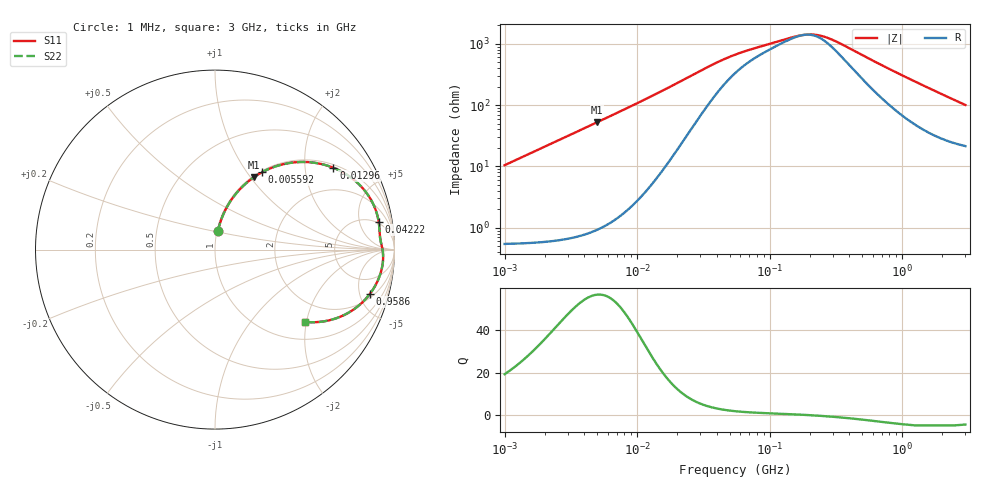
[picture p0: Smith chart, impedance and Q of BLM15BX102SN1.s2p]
! BLM15BX102SN1
# Hz S RI R 50
!Freq.(Hz) S11(Real) S11(Imag) S21(Real) S21(Imag) S12(Real) S12(Imag) S22(Real) S22(Imag)
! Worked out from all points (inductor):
!   401 points, 1 MHz to 3 GHz, reference 50 ohm
!   read as one part in series: L = 1.66 uH near 1.041 MHz
!   highest Q = 56.7 at 4.959 MHz (marker M1), where L = 1.67 uH
!   self-resonance near 183.5 MHz
!   S11 on the Smith chart (normalised r, x): 1 MHz: 1.01, +0.21; 5.592 MHz: 1.02, +1.18; 12.96 MHz: 1.10, +2.82; 42.22 MHz: 5, +10; 958.6 MHz: 2.45, -6.22; 3 GHz: 1.43, -1.96
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1000000  0.016 0.1021  0.984 -0.1021  0.984 -0.1021  0.016 0.1021
2182827  0.0545 0.2143  0.9455 -0.2143  0.9455 -0.2143  0.0545 0.2143
3823119  0.1428 0.3407  0.8572 -0.3407  0.8572 -0.3407  0.1428 0.3407
4959344  0.2175 0.4038  0.7825 -0.4038  0.7825 -0.4038  0.2175 0.4038
5592179  0.2608 0.4303  0.7392 -0.4303  0.7392 -0.4303  0.2608 0.4303
8686058  0.4616 0.4876  0.5384 -0.4876  0.5384 -0.4876  0.4616 0.4876
1.29622e7  0.6599 0.4558  0.3401 -0.4558  0.3401 -0.4558  0.6599 0.4558
1.461624e7  0.7121 0.431  0.2879 -0.431  0.2879 -0.431  0.7121 0.431
1.858443e7  0.7981 0.3678  0.2019 -0.3678  0.2019 -0.3678  0.7981 0.3678
2.362996e7  0.8571 0.2972  0.1429 -0.2972  0.1429 -0.2972  0.8571 0.2972
4.22235e7  0.9121 0.1534  0.0879 -0.1534  0.0879 -0.1534  0.9121 0.1534
5.477226e7  0.9164 0.1114  0.0836 -0.1114  0.0836 -0.1114  0.9164 0.1114
1.460522e8  0.9293 0.0199  0.0707 -0.0199  0.0707 -0.0199  0.9293 0.0199
2.094008e8  0.9351 -0.0125  0.0649 0.0125  0.0649 0.0125  0.9351 -0.0125
2.457655e8  0.9365 -0.0288  0.0635 0.0288  0.0635 0.0288  0.9365 -0.0288
3.002264e8  0.9366 -0.0513  0.0634 0.0513  0.0634 0.0513  0.9366 -0.0513
5.154121e8  0.924 -0.1266  0.076 0.1266  0.076 0.1266  0.924 -0.1266
8.005644e8  0.8889 -0.2079  0.1111 0.2079  0.1111 0.2079  0.8889 -0.2079
9.585869e8  0.8638 -0.2458  0.1362 0.2458  0.1362 0.2458  0.8638 -0.2458
1.347129e9  0.7919 -0.3192  0.2081 0.3192  0.2081 0.3192  0.7919 -0.3192
1.893158e9  0.6842 -0.3795  0.3158 0.3795  0.3158 0.3795  0.6842 -0.3795
3e9  0.501 -0.4024  0.499 0.4024  0.499 0.4024  0.501 -0.4024
